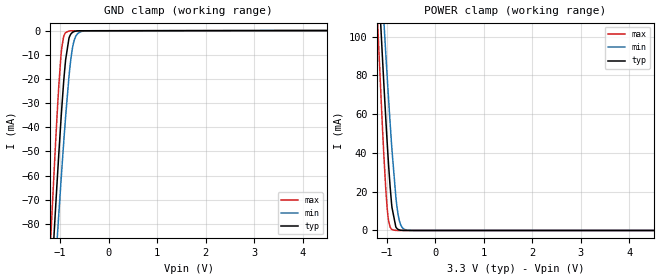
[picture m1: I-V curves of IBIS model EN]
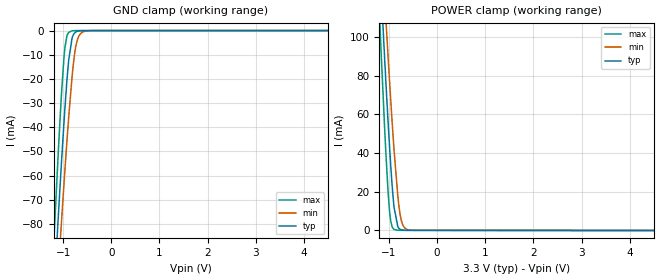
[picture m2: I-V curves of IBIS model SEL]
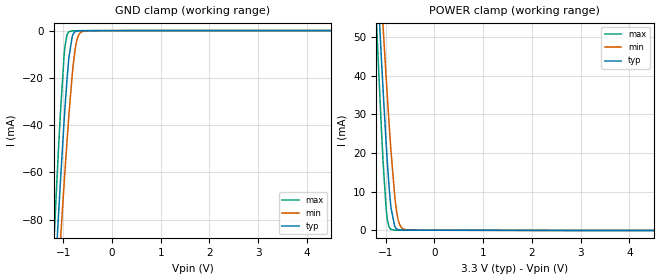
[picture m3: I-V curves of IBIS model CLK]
| Texas Instruments Incorporated
| Low Skew, 1-to-5, Differential-to-3.3V LVPECL Fanout Buffer
| Marketing part#   Voltage Range   Package-type   #pins/pkg drawing
| LMK00725   3.1V - 3.5V   TSSOP   20/PW
[IBIS Ver]   4.1
[File name]   lmk00725.ibs
[File Rev]   1.0
[Date]   06/11/2013
[Source]   Model built from spectre simulations at:
   Texas Instruments Incorporated.
   Analog-eLab, HPA
   12500 TI Blvd
   Dallas, TX -75243
   For Support e-mail: elab_ibis@list.ti.com
[Notes]   Revision History
   Rev 1.0: 06/11/2013
   - QOUT combined pulldown non-monotonic.
   -LVPECL simulation recommendation:
   It is recommended that a small (1nF or less) AC coupling cap
   be used. Larger values will result in long settling times
   - ccomp values are based on PVT settings:
   MIN: Low Voltage, High Temperature, Weak Process
   TYP: Nominal Voltage, Nominal Temperature, Nominal Process
   MAX: High Voltage, Low Temperature, Fast Process
   - C_comp although listed in numerical order of value are obtained from varying PVT conditions.
   For PVT conditions for each specific value, refer to the buffer description under respective [Model].
   IBIS model user is responsible for using appropriate C_comp to simulate for Signal Integrity.
[Disclaimer]  This model is designed as an aid for customers of Texas Instruments
 TI and its licensors and suppliers make no warranties, either expressed
 or implied, with respect to this  model, including the warranties of
 merchantability or fitness for a particular purpose.
 The model is provided solely on an "as is" basis. The entire risk as to
 its quality and performance is with the customer.
[Copyright] (C)Copyright 2013 Texas Instruments Incorporated.
   All rights reserved.
[Component]   LMK00725PW
[Manufacturer]  Texas Instruments Incorporated
[Package]   |20-pin TSSOP PW package
|   typ   min   max
R_pkg   0   0   0
L_pkg   0   0   0
C_pkg   0   0   0
[Pin]   signal_name   model_name   R_pin   L_pin   C_pin
1   Q0   QOUT   0.31653  3.14288n  0.45390p
2   nQ0   QOUT   0.37741  3.16140n  0.42943p
3   Q1   QOUT   0.34370  2.47224n  0.32523p
4   nQ1   QOUT   0.28830  2.13486n  0.30232p
5   Q2   QOUT   0.24981  1.90327n  0.28534p
6   nQ2   QOUT   0.24988  1.90366n  0.28537p
7   Q3   QOUT   0.28844  2.13574n  0.30240p
8   nQ3   QOUT   0.34390  2.47345n  0.32530p
9   Q4   QOUT   0.37729  3.15779n  0.43025p
10   nQ4   QOUT   0.31651  3.14242n  0.45386p
11   VCC   POWER   0.18956  2.90445n  0.49875p
12   CLK_SEL   SEL   0.35667  3.03990n  0.41819p
13   CLK0   CLK   0.32975  2.39344n  0.31031p
14   nCLK0   nCLK   0.28522  2.12364n  0.29683p
15   VEE   GND   0.25309  1.93124n  0.28500p
16   CLK1   CLK   0.24763  1.89871n  0.28319p
17   nCLK1   nCLK   0.27530  2.06403n  0.29632p
18   VCC   POWER   0.17051  1.98189n  0.34969p
19   CLK_EN   EN   0.35851  3.04829n  0.42093p
20   VCC   POWER   0.19145  2.92781n  0.49969p
[Diff pin]  inv_pin  vdiff  tdelay_typ  tdelay_min  tdelay_max
 1   2   NA   0.0s   0.0s   0.0s
 3   4   NA   0.0s   0.0s   0.0s
 5   6   NA   0.0s   0.0s   0.0s
 7   8   NA   0.0s   0.0s   0.0s
 9   10   NA   0.0s   0.0s   0.0s
13   14   0.15   NA   NA   NA
16   17   0.15   NA   NA   NA
| Models and submodels in the file (5): EN (Input), SEL (Input), CLK (Input), nCLK (Input), QOUT (Output)
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|   Model EN
[Model]   EN
Model_type   Input
Vinl = .8
Vinh = 2
|   typ   min   max
|   (nom PVT)   (fast PVT)   (slow PVT)
C_comp   0.309p   0.301p   0.316p
[Voltage Range]   3.3   3.1   3.5
[Temperature Range]   45   125   -40
[Power Clamp Reference]   3.3   3.1   3.5
[GND Clamp Reference]   0   0   0
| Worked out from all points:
|   GND clamp passes 1 mA (typ) near -0.76 V on its own axis
|   POWER clamp passes 1 mA (typ) near -0.79 V on its own axis
[GND Clamp]
|   Voltage   I(typ)   I(min)   I(max)
-3.3V     -924.3mA   -854.8mA   -1.024A
-1.181V   -105.5mA   -125.6mA   -82.42mA
-1.102V   -77.44mA   -100.2mA   -50.84mA
-1.043V   -57.18mA   -81.66mA   -29.07mA
-973.5mV  -35.11mA   -60.72mA   -9.096mA
-924mV    -21.22mA   -46.48mA   -2.425mA
-884.4mV  -12.17mA   -35.74mA   -840.1uA
-815.1mV  -3.203mA   -19.2mA    -159.6uA
-755.7mV  -987.5uA   -8.866mA   -89.6uA
-706.2mV  -384.8uA   -3.987mA   -83.86uA
-518.1mV  -76.96uA   -218.7uA   -79.68uA
6.6V      0A         0A         0A
[POWER Clamp]
|   Voltage   I(typ)   I(min)   I(max)
-3.3V     1.278A     1.181A     1.417A
-1.191V   138.3mA    165.3mA    107.9mA
-1.181V   133.4mA    160.8mA    102.3mA
-1.092V   89.87mA    121.3mA    53.91mA
-1.063V   75.94mA    108.5mA    39.17mA
-983.4mV  41.31mA    75.35mA    8.833mA
-894.3mV  11.82mA    41.43mA    459.4uA
-815.1mV  1.844mA    17.46mA    29.46uA
-765.6mV  523.6uA    7.86mA     16.33uA
-706.2mV  97.18uA    2.467mA    14.06uA
-597.3mV  13.61uA    248.8uA    11.84uA
6.6V      0A         0A         0A
|   Model SEL
[Model]   SEL
Model_type   Input
Vinl = .8
Vinh = 2
|   typ   min   max
|   (nom PVT)   (fast PVT)   (slow PVT)
C_comp   0.309p   0.301p   0.316p
[Voltage Range]   3.3   3.1   3.5
[Temperature Range]   45   125   -40
[Power Clamp Reference]   3.3   3.1   3.5
[GND Clamp Reference]   0   0   0
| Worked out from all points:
|   GND clamp passes 1 mA (typ) near -0.76 V on its own axis
|   POWER clamp passes 1 mA (typ) near -0.79 V on its own axis
[GND Clamp]
|   Voltage   I(typ)   I(min)   I(max)
-3.3V     -924.2mA   -854.8mA   -1.024A
-1.181V   -105.5mA   -125.5mA   -82.35mA
-1.102V   -77.37mA   -100.2mA   -50.77mA
-1.043V   -57.12mA   -81.6mA    -29mA
-973.5mV  -35.04mA   -60.66mA   -9.026mA
-924mV    -21.16mA   -46.42mA   -2.356mA
-884.4mV  -12.1mA    -35.68mA   -770.7uA
-815.1mV  -3.137mA   -19.14mA   -90.22uA
-755.7mV  -921.7uA   -8.805mA   -20.2uA
-706.2mV  -319uA     -3.926mA   -14.46uA
-508.2mV  -10.71uA   -130.8uA   -10.08uA
6.6V      0A         0A         0A
[POWER Clamp]
|   Voltage   I(typ)   I(min)   I(max)
-3.3V     1.278A     1.181A     1.417A
-1.191V   138.4mA    165.4mA    108mA
-1.181V   133.4mA    160.9mA    102.4mA
-1.092V   89.93mA    121.4mA    53.98mA
-1.063V   76mA       108.5mA    39.24mA
-983.4mV  41.38mA    75.41mA    8.903mA
-894.3mV  11.89mA    41.49mA    528.9uA
-815.1mV  1.91mA     17.52mA    98.91uA
-765.6mV  589.4uA    7.92mA     85.77uA
-706.2mV  163uA      2.528mA    83.5uA
-597.3mV  79.45uA    309.5uA    81.28uA
6.6V      0A         0A         0A
|   Model CLK
[Model]   CLK
Model_type   Input
Vinl = 1.2
Vinh = 1.5
|   typ   min   max
|   (nom PVT)   (fast PVT)   (slow PVT)
C_comp   0.302p   0.289p   0.313p
[Voltage Range]   3.3   3.1   3.5
[Temperature Range]   45   125   -40
[Power Clamp Reference]   3.3   3.1   3.5
[GND Clamp Reference]   0   0   0
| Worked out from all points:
|   GND clamp passes 1 mA (typ) near -0.78 V on its own axis
|   POWER clamp passes 1 mA (typ) near -0.82 V on its own axis
[GND Clamp]
|   Voltage   I(typ)   I(min)   I(max)
-3.3V     -971.5mA   -905.8mA   -1.073A
-1.181V   -109mA     -130.1mA   -84.92mA
-1.102V   -79.56mA   -103.4mA   -51.85mA
-1.063V   -65.29mA   -90.37mA   -36.37mA
-973.5mV  -35.21mA   -61.93mA   -8.387mA
-924mV    -20.73mA   -47mA      -1.789mA
-884.4mV  -11.36mA   -35.75mA   -487.3uA
-815.1mV  -2.39mA    -18.5mA    -89.58uA
-745.8mV  -413.2uA   -6.606mA   -52.22uA
-676.5mV  -94.57uA   -1.625mA   -47.63uA
-577.5mV  -48.53uA   -211uA     -43.69uA
6.6V      0A         0A         0A
[POWER Clamp]
|   Voltage   I(typ)   I(min)   I(max)
-3.3V     640.7mA    598mA      708.5mA
-1.191V   69.24mA    82.72mA    54.05mA
-1.181V   66.77mA    80.49mA    51.25mA
-1.092V   45.01mA    60.74mA    27.03mA
-1.053V   35.77mA    52.19mA    17.34mA
-973.5mV  18.76mA    35.75mA    3.394mA
-894.3mV  5.987mA    20.78mA    307.9uA
-815.1mV  996.1uA    8.797mA    92.17uA
-765.6mV  335.2uA    3.998mA    85.11uA
-706.2mV  121.4uA    1.301mA    83.39uA
-607.2mV  79.09uA    223uA      81.4uA
6.6V      0A         0A         0A
